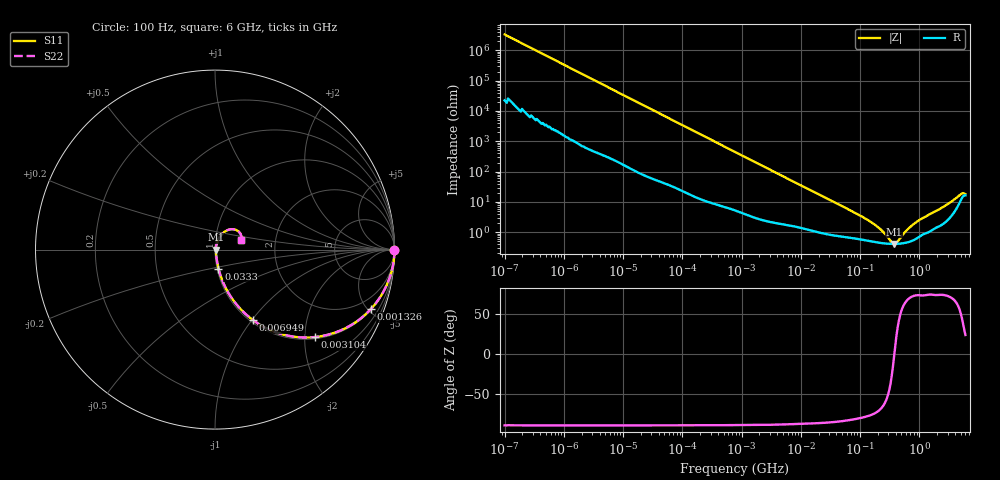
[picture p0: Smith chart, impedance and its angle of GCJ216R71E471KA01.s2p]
!Murata Part Number: GCJ216R71E471KA01
!These Parameters are Measured in Series Mode Connection
!Data Generated on Mar 13, 2026
!  o--ll--o
!Port1  Port2
!  o------o
!Operation Temp=25[degC], DC Bias Voltage=0[V]
!Freq. Start=100[Hz] Stop=6[GHz] 401[Steps]
# Hz S RI R 50
!Freq.(Hz) S11(Real) S11(Imag) S21(Real) S21(Imag) S12(Real) S12(Imag) S22(Real) S22(Imag)
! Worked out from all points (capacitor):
!   401 points, 100 Hz to 6 GHz, reference 50 ohm
!   read as one part in series: C = 473 pF near 109 Hz
!   lowest |Z| = 414 mohm at 373.7 MHz (marker M1)
!   series resonance near 379.4 MHz, so ESL is about 370 pH
!   S11 on the Smith chart (normalised r, x): 100 Hz: open; 1.326 MHz: 1.07, -5.25; 3.104 MHz: 1.04, -2.25; 6.949 MHz: 1.03, -1.01; 33.3 MHz: 1.02, -0.22; 6 GHz: 1.33, +0.15
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100  1 -2.98e-05  2e-07 2.98e-05  2e-07 2.98e-05  1 -2.98e-05
350  1 -0.000104  6e-07 0.000104  6e-07 0.000104  1 -0.000104
2008  1 -0.000592  2.8e-06 0.000592  2.8e-06 0.000592  1 -0.000592
40335  0.9998 -0.0118  0.000206 0.0118  0.000206 0.0118  0.9998 -0.0118
241822  0.9946 -0.0698  0.00543 0.0698  0.00543 0.0698  0.9946 -0.0698
774597  0.9501 -0.2118  0.0499 0.2118  0.0499 0.2118  0.9501 -0.2118
1325623  0.8698 -0.3298  0.1302 0.3298  0.1302 0.3298  0.8698 -0.3298
1983483  0.7521 -0.4242  0.2479 0.4242  0.2479 0.4242  0.7521 -0.4242
3103719  0.558 -0.4871  0.442 0.4871  0.442 0.4871  0.558 -0.4871
6948629  0.2121 -0.3931  0.7879 0.3931  0.7879 0.3931  0.2121 -0.3931
1.555665e7  0.0596 -0.2137  0.9404 0.2137  0.9404 0.2137  0.0596 -0.2137
3.330331e7  0.0193 -0.1053  0.9807 0.1053  0.9807 0.1053  0.0193 -0.1053
1.596157e8  0.00532 -0.0198  0.9947 0.0198  0.9947 0.0198  0.00532 -0.0198
2.283698e8  0.00452 -0.0109  0.9955 0.0109  0.9955 0.0109  0.00452 -0.0109
3.124326e8  0.00416 -0.00408  0.9958 0.00408  0.9958 0.00408  0.00416 -0.00408
3.737127e8  0.00411 -0.000315  0.9959 0.000315  0.9959 0.000315  0.00411 -0.000315
4.274388e8  0.00415 0.00252  0.9959 -0.00252  0.9959 -0.00252  0.00415 0.00252
6.395615e8  0.0048 0.0116  0.9952 -0.0116  0.9952 -0.0116  0.0048 0.0116
9.569533e8  0.00718 0.0226  0.9928 -0.0226  0.9928 -0.0226  0.00718 0.0226
2.931063e9  0.029 0.0742  0.971 -0.0742  0.971 -0.0742  0.029 0.0742
4.796499e9  0.1012 0.1135  0.8988 -0.1135  0.8988 -0.1135  0.1012 0.1135
6e9  0.1456 0.0534  0.8544 -0.0534  0.8544 -0.0534  0.1456 0.0534
